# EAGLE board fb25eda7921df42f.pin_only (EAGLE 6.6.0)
REV: B

Size 65 x 56.5 mm. Coordinates in mm from the lower left corner, seen from the top.
Copper layers (1*16): Top 0.035mm / dielectric 1.5mm / Bottom 0.035mm
Design rules "adafruit": minimum track width 8mil, minimum drill 15.5mil, track to track 8mil, track to pad 8mil, pad to pad 8mil, via to via 8mil, smd to smd 8mil, copper to edge 10mil, drill to drill 8mil, minimum pad ring 10mil, minimum via ring 8mil, stop-mask expansion 4mil, vias tented up to drill 20mil, thermal gap 10mil

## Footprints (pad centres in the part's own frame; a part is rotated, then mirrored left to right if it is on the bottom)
0805-NO = smd 1.3 x 1.5: 1 -0.95,0; 2 0.95,0
_0805MP = smd 1.2 x 1.3: 1 -1.016,0; 2 1.016,0
SMADIODE = smd 2.54 x 2.54: A 2.349,0; C -2.349,0
SOD-123 = smd 1.4 x 1.4: A 1.85,0; C -1.85,0
SOD-323 = smd 1.35 x 0.8: A 1.27,0; C -1.27,0
FIDUCIAL_1MM = smd 1 x 1: 1 0,0
TSSOP20-5.3MMBODY = smd 0.305 x 1.27: 1 -2.925,-3.618; 2 -2.275,-3.618; 3 -1.625,-3.618; 4 -0.975,-3.618; 5 -0.325,-3.618; 6 0.325,-3.618; 7 0.975,-3.618; 8 1.625,-3.618; 9 2.275,-3.618; 10 2.925,-3.618; 11 2.925,3.618; 12 2.275,3.618; 13 1.625,3.618; 14 0.975,3.618; 15 0.325,3.618; 16 -0.325,3.618; 17 -0.975,3.618; 18 -1.625,3.618; 19 -2.275,3.618; 20 -2.925,3.618
4-1734839-0 = smd 0.25 x 1.1: 1 -9.75,-2.54; 2 -9.25,-2.54; 3 -8.75,-2.54; 4 -8.25,-2.54; 5 -7.75,-2.54; 6 -7.25,-2.54; 7 -6.75,-2.54; 8 -6.25,-2.54; 9 -5.75,-2.54; 10 -5.25,-2.54; 11 -4.75,-2.54; 12 -4.25,-2.54; 13 -3.75,-2.54; 14 -3.25,-2.54; 15 -2.75,-2.54; 16 -2.25,-2.54; 17 -1.75,-2.54; 18 -1.25,-2.54; 19 -0.75,-2.54; 20 -0.25,-2.54; 21 0.25,-2.54; 22 0.75,-2.54; 23 1.25,-2.54; 24 1.75,-2.54; 25 2.25,-2.54; 26 2.75,-2.54; 27 3.25,-2.54; 28 3.75,-2.54; 29 4.25,-2.54; 30 4.75,-2.54; 31 5.25,-2.54; 32 5.75,-2.54; 33 6.25,-2.54; 34 6.75,-2.54; 35 7.25,-2.54; 36 7.75,-2.54; 37 8.25,-2.54; 38 8.75,-2.54; 39 9.25,-2.54; 40 9.75,-2.54 | smd 2.3 x 3.1: M1 11.4,-0.84; M2 -11.4,-0.84
INDUCTOR_5X5MM_NR5040_NOTHERMALS = smd 1.8 x 4: P$1 -1.8,0; P$2 1.8,0
CHIPLED_0805_NOOUTLINE = smd 1.2 x 1.2: A 0,-1.05; C 0,1.05
RESPACK_4X0603 = smd 0.45 x 0.9: 1 -1.3,-0.85; 2 -0.4,-0.85; 3 0.4,-0.85; 4 1.3,-0.85; 5 1.3,0.85; 6 0.4,0.85; 7 -0.4,0.85; 8 -1.3,0.85
PI_HAT_SMT_SLOTS = smd 1.524 x 3.048 bottom: 1 8.395,50.349; 2 8.395,54.667; 3 10.935,50.349; 4 10.935,54.667; 5 13.475,50.349; 6 13.475,54.667; 7 16.015,50.349; 8 16.015,54.667; 9 18.555,50.349; 10 18.555,54.667; 11 21.095,50.349; 12 21.095,54.667; 13 23.635,50.349; 14 23.635,54.667; 15 26.175,50.349; 16 26.175,54.667; 17 28.715,50.349; 18 28.715,54.667; 19 31.255,50.349; 20 31.255,54.667; 21 33.795,50.349; 22 33.795,54.667; 23 36.335,50.349; 24 36.335,54.667; 25 38.875,50.349; 26 38.875,54.667; 27 41.415,50.349; 28 41.415,54.667; 29 43.955,50.349; 30 43.955,54.667; 31 46.495,50.349; 32 46.495,54.667; 33 49.035,50.349; 34 49.035,54.667; 35 51.575,50.349; 36 51.575,54.667; 37 54.115,50.349; 38 54.115,54.667; 39 56.655,50.349; 40 56.655,54.667 | hole 2.8: 3.5,3.5; 3.5,52.5; 61.5,52.5; 61.5,3.5
SOLDERJUMPER_ARROW_NOPASTE = smd 0.762 x 1.524: 1 -1.016,0; 2 1.016,0
TP15SQ = smd 1.5 x 1.5: TP 0,0
SOT23-5@1 = smd 0.55 x 1.2: 1 -0.95,-1.3; 2 0,-1.3; 3 0.95,-1.3; 4 0.95,1.3; 5 -0.95,1.3
4UCONN_20329 = smd 1 x 2: BASE@1 -0.75,-2; BASE@2 0.75,-2 | smd 0.4 x 1.35: D+ 0,0.775; D- -0.65,0.775; GND 1.3,0.775; ID 0.65,0.775; VBUS -1.3,0.775 | drill 0.7 offset: SPRT@1 -3.3,0.9; SPRT@2 3.3,0.9 | drill 0.6 pad 2.5 square: SPRT@3 -3.6,-1.9; SPRT@4 3.6,-1.9 | hole 0.7: -1.95,0; 1.95,0
RESONATOR-SMD = smd 0.7 x 1.7: 1 -1.2,0; 2 0,0; 3 1.2,0

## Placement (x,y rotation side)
C1  0.1uF  [0805-NO]  8,36.94 0 top
C2  1uF  [_0805MP]  14.99,45.58 270 top
C3  0.1uF  [0805-NO]  47.88,43.16 270 top
C4  10uF  [0805-NO]  56.77,49.52 0 top
C5  10uF  [0805-NO]  59.56,43.8 270 top
C7  10uF  [0805-NO]  9.4,29.2 180 top
C8  1uF  [0805-NO]  11.56,36.94 180 top
D1  MM3Z24VT1G  [SMADIODE]  9.91,49.01 180 top
D2  MBR0540  [SOD-123]  15.11,37.83 270 top
D3  1N4148  [SOD-323]  8.51,24.88 90 top
FB1  FERRITE  [_0805MP]  57.02,35.67 270 top
FB2  FERRITE  [_0805MP]  54.74,35.67 270 top
FB3  Ferrite  [_0805MP]  50.16,35.67 270 top
FB4  FERITE  [_0805MP]  52.32,35.67 270 top
FID1  FIDUCIAL""  [FIDUCIAL_1MM]  59.69,1.38 0 top
FID2  FIDUCIAL""  [FIDUCIAL_1MM]  2.29,6.97 0 top
FID3  FIDUCIAL""  [FIDUCIAL_1MM]  6.1,54.72 0 top
IC1  AR1100_SSOP  [TSSOP20-5.3MMBODY]  53.85,44.31 270 top
J1  40PINFPCM4-1734839-0  [4-1734839-0]  28.96,52.69 0 top
L1  6.8uH power L CID 2276  [INDUCTOR_5X5MM_NR5040_NOTHERMALS]  13.97,32.12 90 top
LED1  RED  [CHIPLED_0805_NOOUTLINE]  63.25,46.47 180 top
R1  20K  [0805-NO]  9.4,30.97 0 top
R2  6Ω  [0805-NO]  11.68,42.53 0 top
R3  12Ω  [0805-NO]  4.57,42.53 0 top
R4  12Ω  [0805-NO]  8.13,42.53 0 top
R5  20K  [_0805MP]  14.86,54.21 270 top
R6  33  [RESPACK_4X0603]  19.05,44.56 180 top
R7  12Ω  [0805-NO]  11.56,38.72 0 top
R8  33  [RESPACK_4X0603]  23.11,44.56 0 top
R9  33  [RESPACK_4X0603]  27.18,44.56 0 top
R10  33  [RESPACK_4X0603]  31.24,44.56 0 top
R11  33  [RESPACK_4X0603]  35.31,44.56 0 top
R12  33  [RESPACK_4X0603]  39.37,44.56 0 top
R13  470  [0805-NO]  63.25,42.53 90 top
R14  20K  [0805-NO]  58.04,39.86 0 top
RPI1  RASPBERRYPI_BPLUS-SMT+SLOTS  [PI_HAT_SMT_SLOTS]  0,56.5 180 bottom
SJ1  +50mA  [SOLDERJUMPER_ARROW_NOPASTE]  11.68,44.56 180 top
SJ2  +25mA  [SOLDERJUMPER_ARROW_NOPASTE]  4.57,44.56 180 top
SJ3  +100mA  [SOLDERJUMPER_ARROW_NOPASTE]  8.13,44.56 180 top
TP1  TPTP15SQ  [TP15SQ]  24.38,15.1 0 top
TP2  TPTP15SQ  [TP15SQ]  26.92,15.1 0 top
TP3  TPTP15SQ  [TP15SQ]  29.46,15.1 0 top
TP4  TPTP15SQ  [TP15SQ]  32,15.1 0 top
TP5  TPTP15SQ  [TP15SQ]  6.6,15.1 0 top
TP6  TPTP15SQ  [TP15SQ]  9.14,15.1 0 top
TP7  TPTP15SQ  [TP15SQ]  11.68,15.1 0 top
TP8  TPTP15SQ  [TP15SQ]  14.22,15.1 0 top
TP9  TPTP15SQ  [TP15SQ]  16.76,15.1 0 top
TP10  TPTP15SQ  [TP15SQ]  21.84,15.1 0 top
TP11  TPTP15SQ  [TP15SQ]  19.3,15.1 0 top
TP12  TPTP15SQ  [TP15SQ]  34.54,15.1 0 top
TP13  TPTP15SQ  [TP15SQ]  54.86,15.1 0 top
U3  FAN5333BSX  [SOT23-5@1]  9.4,33.89 180 top
U$30  [ADAFRUIT_TEXT_30MM]  17.91,24.5 0 top
U$31  [ADAFRUIT_TEXT_30MM]  47.24,26.02 0 bottom
U$32  [PCBFEAT-REV-040]  52.45,21.83 0 top
X1  MicroUSB  [4UCONN_20329]  52.7,52.18 180 top
Y1  12MHz  [RESONATOR-SMD]  47.75,47.1 270 top

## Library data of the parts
C1-C5 C7 C8 D1-D3 FB1-FB4 IC1 L1 LED1 R1-R14 RPI1 U3 U$30-U$32 X1 = microbuilder
FID1-FID3 SJ1-SJ3 = microbuilder; BOM: EXCLUDE
J1 = adafruit
TP1-TP13 = testpad
Y1 = SparkFun

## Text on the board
tPlace: +25mA | +50mA | Backlight: 24V max CC / 25mA-125mA w/jumpers | AR1100 USB Touch | 40-Pin TTL Display Kippah | BACKLIT | On/Off | +5V | +3.3V | GND | GND | GND | #27 | #22 | #23 | #24 | #25 | #26
bPlace: Connect standard 40-pin / DPI / DotClock type Display | Opt. USB / Mouse / Touchscreen | Adjust constant-current / backlight by soldering / closed jumpers on other side | 40-Pin TTL Display Kippah / (w/optional touch screen control) | Note: Replaces the HDMI display out | Note: Uses Pi GPIO pins 2 thru 21

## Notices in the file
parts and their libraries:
SparkFun: Licensing: CC v3.0 Share-Alike You are welcome to use this library for commercial purposes.
